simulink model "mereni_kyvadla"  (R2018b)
settings: Solver=ode4  StartTime=0.0  StopTime=inf  FixedStep=1e-3  RelTol=1e-3
undefined symbols (not defined in the file or in its folder): Humusoft, MF624
libraries: simulink x2, sldrtlib x2

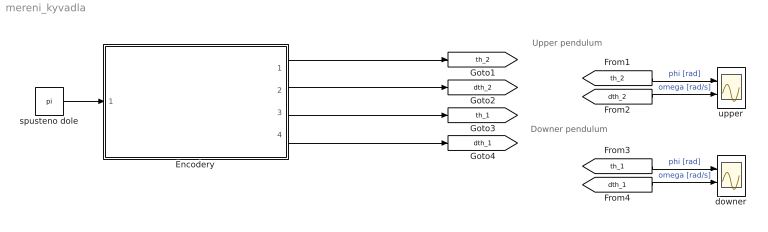
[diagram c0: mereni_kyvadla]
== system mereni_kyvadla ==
  note: Downer pendulum
  note: Upper pendulum
  Encodery : Subsystem
  downer : Scope  NumInputPorts=2
  spusteno dole : Constant  Value=pi
  upper : Scope  NumInputPorts=2
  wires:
  Encodery/1(th2 [rad]) -> [th_2]
  Encodery/3(th1 [rad]) -> [th_1]
  Encodery/2(dth2 [rad/s]) -> [dth_2]
  Encodery/4(dth1 [rad/s]) -> [dth_1]
  [th_1] -> downer/1  "phi [rad]"
  [dth_1] -> downer/2  "omega [rad/s]"
  [dth_2] -> upper/2  "omega [rad/s]"
  [th_2] -> upper/1  "phi [rad]"
  spusteno dole/1 -> Encodery/1(pocatecni poloha [rad])

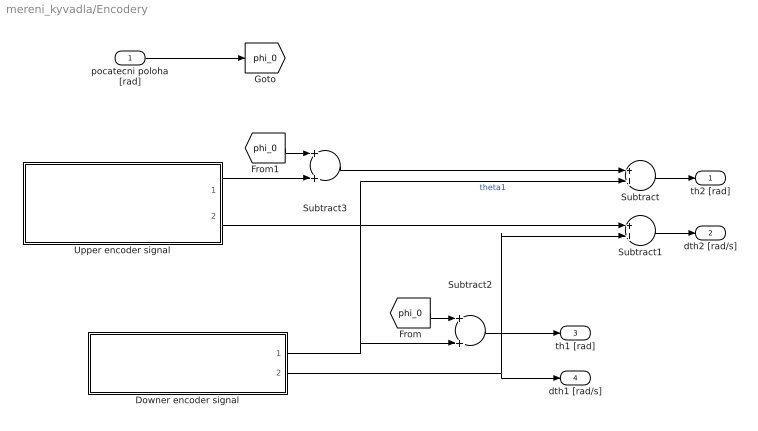
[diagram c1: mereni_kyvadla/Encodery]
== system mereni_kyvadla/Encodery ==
  pocatecni poloha [rad] : Inport
  Downer encoder signal : Subsystem
  Subtract{,1..3} (4 alike) : Sum
  Upper encoder signal : Subsystem
  th2 [rad] : Outport
  dth2 [rad/s] : Outport  Port=2
  th1 [rad] : Outport  Port=3
  dth1 [rad/s] : Outport  Port=4
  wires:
  Downer encoder signal/2(omega [rad/s]) -> Subtract1/2, dth1 [rad/s]/1
  Subtract/1 -> th2 [rad]/1
  Subtract1/1 -> dth2 [rad/s]/1
  Upper encoder signal/2(omega [rad/s]) -> Subtract1/1
  Downer encoder signal/1(phi [rad]) -> Subtract/2, Subtract2/2  "theta1"
  Subtract2/1 -> th1 [rad]/1
  pocatecni poloha [rad]/1 -> [phi_0]
  [phi_0] -> Subtract2/1
  Upper encoder signal/1(phi [rad]) -> Subtract3/2
  [phi_0] -> Subtract3/1
  Subtract3/1 -> Subtract/1

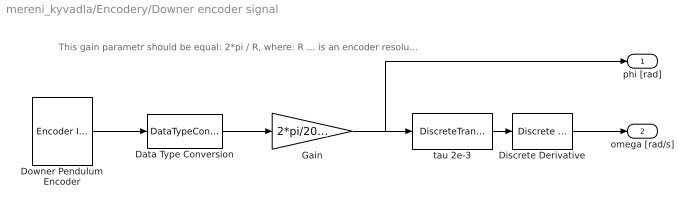
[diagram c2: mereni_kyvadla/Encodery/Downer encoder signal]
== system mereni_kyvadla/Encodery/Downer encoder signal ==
  note: This gain parametr should be equal: 2*pi / R, where: R ... is an encoder resolution
  Data Type Conversion : DataTypeConversion  OutDataTypeStr=double
  Discrete Derivative : simulink/Discrete/Discrete Derivative  gainval=1.0  ICPrevScaledInput=0.0  OutMin=[]  OutMax=[]  OutDataType=fixdt(1, 16)  OutScaling=2^-10  DoSatur=off
  Downer Pendulum Encoder : sldrtlib/Encoder Input  SampleTime=0.001  MaxMissedTicks=1e6  ShowMissedTicks=off  YieldWhenWaiting=off  DrvName=Humusoft/MF624  DrvAddress=4294967295  DrvOptions=0  Channels=2  QuadMode=3  IndexPulse=1  InputFilter=Inf  DataType=7
  Gain : Gain  Gain=2*pi/2048
  tau 2e-3 : DiscreteTransferFcn  Numerator=0.3935  Denominator=[1 -0.6065]
  phi [rad] : Outport
  omega [rad/s] : Outport  Port=2
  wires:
  Downer Pendulum Encoder/1 -> Data Type Conversion/1
  Discrete Derivative/1 -> omega [rad/s]/1
  Data Type Conversion/1 -> Gain/1
  Gain/1 -> tau 2e-3/1, phi [rad]/1
  tau 2e-3/1 -> Discrete Derivative/1

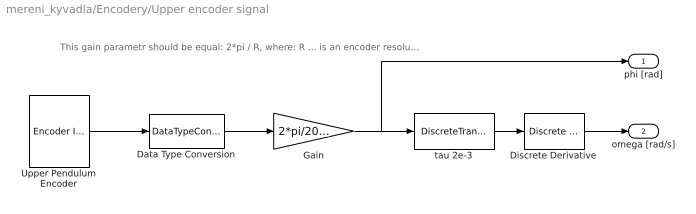
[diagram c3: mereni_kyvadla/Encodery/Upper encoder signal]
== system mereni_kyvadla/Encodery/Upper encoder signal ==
  note: This gain parametr should be equal: 2*pi / R, where: R ... is an encoder resolution
  Data Type Conversion : DataTypeConversion  OutDataTypeStr=double
  Discrete Derivative : simulink/Discrete/Discrete Derivative  gainval=1.0  ICPrevScaledInput=0.0  OutMin=[]  OutMax=[]  OutDataType=fixdt(1, 16)  OutScaling=2^-10  DoSatur=off
  Gain : Gain  Gain=2*pi/2048
  Upper Pendulum Encoder : sldrtlib/Encoder Input  SampleTime=0.001  MaxMissedTicks=1e6  ShowMissedTicks=off  YieldWhenWaiting=off  DrvName=Humusoft/MF624  DrvAddress=4294967295  DrvOptions=0  Channels=4  QuadMode=3  IndexPulse=1  InputFilter=Inf  DataType=7
  tau 2e-3 : DiscreteTransferFcn  Numerator=0.3935  Denominator=[1 -0.6065]
  phi [rad] : Outport
  omega [rad/s] : Outport  Port=2
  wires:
  Upper Pendulum Encoder/1 -> Data Type Conversion/1
  Discrete Derivative/1 -> omega [rad/s]/1
  Data Type Conversion/1 -> Gain/1
  Gain/1 -> tau 2e-3/1, phi [rad]/1
  tau 2e-3/1 -> Discrete Derivative/1
